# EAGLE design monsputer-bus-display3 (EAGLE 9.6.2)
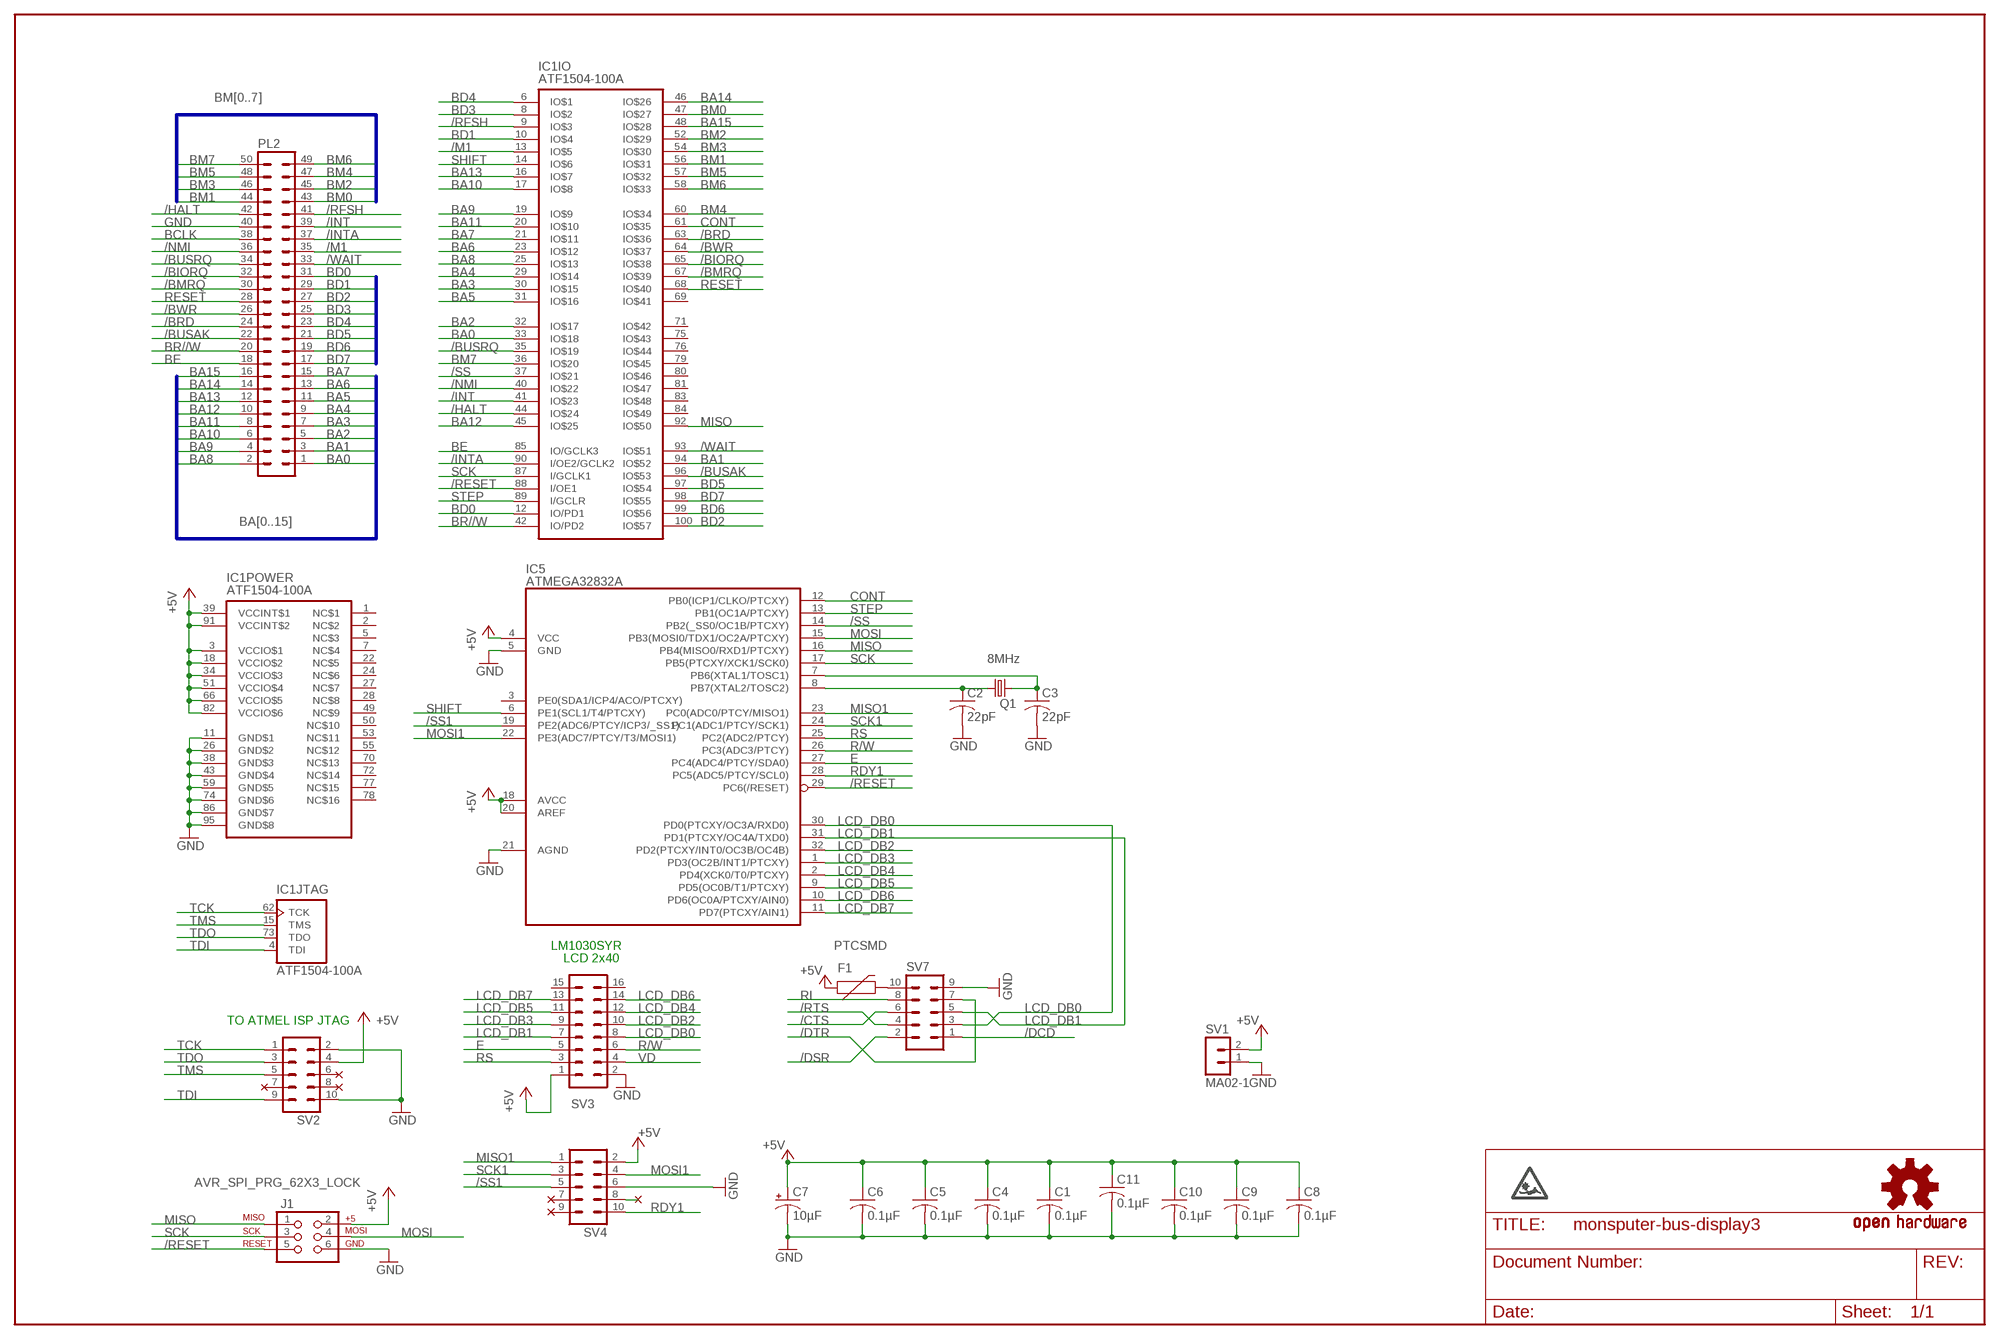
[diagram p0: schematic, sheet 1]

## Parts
C1  0.1µF  C-USC0603  [C0603]
C2  22pF  C-USC0603  [C0603]
C3  22pF  C-USC0603  [C0603]
C4  0.1µF  C-USC0603  [C0603]
C5  0.1µF  C-USC0603  [C0603]
C6  0.1µF  C-USC0603  [C0603]
C7  10µF  CPOL-USCT3528  [CT3528]
C8  0.1µF  C-USC0603  [C0603]
C9  0.1µF  C-USC0603  [C0603]
C10  0.1µF  C-USC0603  [C0603]
C11  0.1µF  C-USC0603  [C0603]
F1  PTCSMD  [PTC-1206]
IC1  ATF1504-100A  [TQFP100]
IC5  ATMEGA32832A  [TQFP32-08]
J1  AVR_SPI_PRG_62X3_LOCK  [2X3_LOCK]
PL2  50H  [50H]
Q1  8MHz  CRYSTALHC49US  [HC49US]
SV1  MA02-1  [MA02-1]
SV2  MA05-2  [MA05-2]
SV3  MA08-2  [MA08-2]
SV4  MA05-2  [MA05-2]
SV7  MA05-2  [MA05-2]
U$1  PHYSNOCT  [PHYSNOCT]
U$2  OSHW-LOGOS  [OSHW-LOGO-S]

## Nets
+5V: C1.1 C4.1 C5.1 C6.1 C7.+ C8.1 C9.1 C10.1 C11.1 F1.1 IC1.3(POWER:VCCIO$1) IC1.18(POWER:VCCIO$2) IC1.34(POWER:VCCIO$3) IC1.39(POWER:VCCINT$1) IC1.51(POWER:VCCIO$4) IC1.66(POWER:VCCIO$5) IC1.82(POWER:VCCIO$6) IC1.91(POWER:VCCINT$2) IC5.4(VCC) IC5.18(AVCC) IC5.20(AREF) J1.2 SV1.2 SV2.4 SV3.1 SV4.2
/BIORQ: IC1.65(IO:IO$38) PL2.32
/BMRQ: IC1.67(IO:IO$39) PL2.30
/BRD: IC1.63(IO:IO$36) PL2.24
/BUSAK: IC1.96(IO:IO$53) PL2.22
/BUSRQ: IC1.35(IO:IO$19) PL2.34
/BWR: IC1.64(IO:IO$37) PL2.26
/CTS: SV7.6
/DCD: SV7.1
/DSR: SV7.2
/DTR: SV7.7
/HALT: IC1.44(IO:IO$24) PL2.42
/INT: IC1.41(IO:IO$23) PL2.39
/INTA: IC1.90(IO:I/OE2/GCLK2) PL2.37
/M1: IC1.13(IO:IO$5) PL2.35
/NMI: IC1.40(IO:IO$22) PL2.36
/RESET: IC1.88(IO:I/OE1) IC5.29(PC6(/RESET)) J1.5
/RFSH: IC1.9(IO:IO$3) PL2.41
/RTS: SV7.4
/SS: IC1.37(IO:IO$21) IC5.14(PB2(_SS0/OC1B/PTCXY))
/SS1: IC5.19(PE2(ADC6/PTCY/ICP3/_SS1)) SV4.5
/WAIT: IC1.93(IO:IO$51) PL2.33
BA0: IC1.33(IO:IO$18) PL2.1
BA1: IC1.94(IO:IO$52) PL2.3
BA2: IC1.32(IO:IO$17) PL2.5
BA3: IC1.30(IO:IO$15) PL2.7
BA4: IC1.29(IO:IO$14) PL2.9
BA5: IC1.31(IO:IO$16) PL2.11
BA6: IC1.23(IO:IO$12) PL2.13
BA7: IC1.21(IO:IO$11) PL2.15
BA8: IC1.25(IO:IO$13) PL2.2
BA9: IC1.19(IO:IO$9) PL2.4
BA10: IC1.17(IO:IO$8) PL2.6
BA11: IC1.20(IO:IO$10) PL2.8
BA12: IC1.45(IO:IO$25) PL2.10
BA13: IC1.16(IO:IO$7) PL2.12
BA14: IC1.46(IO:IO$26) PL2.14
BA15: IC1.48(IO:IO$28) PL2.16
BCLK: PL2.38
BD0: IC1.12(IO:IO/PD1) PL2.31
BD1: IC1.10(IO:IO$4) PL2.29
BD2: IC1.100(IO:IO$57) PL2.27
BD3: IC1.8(IO:IO$2) PL2.25
BD4: IC1.6(IO:IO$1) PL2.23
BD5: IC1.97(IO:IO$54) PL2.21
BD6: IC1.99(IO:IO$56) PL2.19
BD7: IC1.98(IO:IO$55) PL2.17
BE: IC1.85(IO:IO/GCLK3) PL2.18
BM0: IC1.47(IO:IO$27) PL2.43
BM1: IC1.56(IO:IO$31) PL2.44
BM2: IC1.52(IO:IO$29) PL2.45
BM3: IC1.54(IO:IO$30) PL2.46
BM4: IC1.60(IO:IO$34) PL2.47
BM5: IC1.57(IO:IO$32) PL2.48
BM6: IC1.58(IO:IO$33) PL2.49
BM7: IC1.36(IO:IO$20) PL2.50
BR//W: IC1.42(IO:IO/PD2) PL2.20
CONT: IC1.61(IO:IO$35) IC5.12(PB0(ICP1/CLKO/PTCXY))
E: IC5.27(PC4(ADC4/PTCY/SDA0)) SV3.5
GND: C1.2 C2.2 C3.2 C4.2 C5.2 C6.2 C7.- C8.2 C9.2 C10.2 C11.2 IC1.11(POWER:GND$1) IC1.26(POWER:GND$2) IC1.38(POWER:GND$3) IC1.43(POWER:GND$4) IC1.59(POWER:GND$5) IC1.74(POWER:GND$6) IC1.86(POWER:GND$7) IC1.95(POWER:GND$8) IC5.5(GND) IC5.21(AGND) J1.6 PL2.40 SV1.1 SV2.2 SV2.10 SV3.2 SV4.6 SV7.9
LCD_DB0: IC5.30(PD0(PTCXY/OC3A/RXD0)) SV3.8 SV7.3
LCD_DB1: IC5.31(PD1(PTCXY/OC4A/TXD0)) SV3.7 SV7.5
LCD_DB2: IC5.32(PD2(PTCXY/INT0/OC3B/OC4B)) SV3.10
LCD_DB3: IC5.1(PD3(OC2B/INT1/PTCXY)) SV3.9
LCD_DB4: IC5.2(PD4(XCK0/T0/PTCXY)) SV3.12
LCD_DB5: IC5.9(PD5(OC0B/T1/PTCXY)) SV3.11
LCD_DB6: IC5.10(PD6(OC0A/PTCXY/AIN0)) SV3.14
LCD_DB7: IC5.11(PD7(PTCXY/AIN1)) SV3.13
MISO: IC1.92(IO:IO$50) IC5.16(PB4(MISO0/RXD1/PTCXY)) J1.1
MISO1: IC5.23(PC0(ADC0/PTCY/MISO1)) SV4.1
MOSI: IC5.15(PB3(MOSI0/TDX1/OC2A/PTCXY)) J1.4
MOSI1: IC5.22(PE3(ADC7/PTCY/T3/MOSI1)) SV4.4
N$1: F1.2 SV7.10
N$19: SV4.8
N$20: C3.1 IC5.7(PB6(XTAL1/TOSC1)) Q1.2
N$21: C2.1 IC5.8(PB7(XTAL2/TOSC2)) Q1.1
R/W: IC5.26(PC3(ADC3/PTCY)) SV3.6
RDY1: IC5.28(PC5(ADC5/PTCY/SCL0)) SV4.10
RESET: IC1.68(IO:IO$40) PL2.28
RI: SV7.8
RS: IC5.25(PC2(ADC2/PTCY)) SV3.3
SCK: IC1.87(IO:I/GCLK1) IC5.17(PB5(PTCXY/XCK1/SCK0)) J1.3
SCK1: IC5.24(PC1(ADC1/PTCY/SCK1)) SV4.3
SHIFT: IC1.14(IO:IO$6) IC5.6(PE1(SCL1/T4/PTCXY))
STEP: IC1.89(IO:I/GCLR) IC5.13(PB1(OC1A/PTCXY))
TCK: IC1.62(JTAG:TCK) SV2.1
TDI: IC1.4(JTAG:TDI) SV2.9
TDO: IC1.73(JTAG:TDO) SV2.3
TMS: IC1.15(JTAG:TMS) SV2.5
VD: SV3.4
Unconnected: IC1.1(POWER:NC$1) IC1.2(POWER:NC$2) IC1.5(POWER:NC$3) IC1.7(POWER:NC$4) IC1.22(POWER:NC$5) IC1.24(POWER:NC$6) IC1.27(POWER:NC$7) IC1.28(POWER:NC$8) IC1.49(POWER:NC$9) IC1.50(POWER:NC$10) IC1.53(POWER:NC$11) IC1.55(POWER:NC$12) IC1.69(IO:IO$41) IC1.70(POWER:NC$13) IC1.71(IO:IO$42) IC1.72(POWER:NC$14) IC1.75(IO:IO$43) IC1.76(IO:IO$44) IC1.77(POWER:NC$15) IC1.78(POWER:NC$16) IC1.79(IO:IO$45) IC1.80(IO:IO$46) IC1.81(IO:IO$47) IC1.83(IO:IO$48) IC1.84(IO:IO$49) IC5.3(PE0(SDA1/ICP4/ACO/PTCXY)) SV2.6 SV2.7 SV2.8 SV3.15 SV3.16 SV4.7 SV4.9

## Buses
BD[0..7]
BM[0..7]
BA[0..15]

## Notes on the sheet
- LM1030SYR
- LCD 2x40
- TO ATMEL ISP JTAG

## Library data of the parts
C1-C6 C8-C11 = rcl:C-US: CAPACITOR, American symbol
C7 = rcl:CPOL-US: POLARIZED CAPACITOR, American symbol
F1 = SparkFun:PTC: Resettable Fuse PTC
IC1 = newchips:ATF1504-100: Atmel 64-macrocell CPLD
IC5 = newchips2:ATMEGA328: ATmega328PB AVR® Microcontroller with Core Independent Peripherals and PicoPower® Technology
J1 = SparkFun:AVR_SPI_PRG_6: AVR ISP 6 Pin This is the reduced ISP connector for AVR programming. Common on Arduino. This footprint will take up less PCB space and can be used with a 10-pin to 6-pin adapter such as SKU: BOB-08508
PL2 = con-harting-h:50H: CONNECTOR
Q1 = SparkFun:CRYSTAL: Crystals
SV1 = divers:MA02-1: PIN HEADER
SV2 SV4 SV7 = con-lstb:MA05-2: PIN HEADER; OC_FARNELL: unknown; OC_NEWARK: unknown
SV3 = con-lstb:MA08-2: PIN HEADER; OC_FARNELL: unknown; OC_NEWARK: unknown
U$1 = physnoct:PHYSNOCT: Physnoct logo
U$2 = SparkFun:OSHW-LOGO: Open Source Hardware Logo This logo indicates the piece of hardware it is found on incorporates a OSHW license and/or adheres to the definition of open source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

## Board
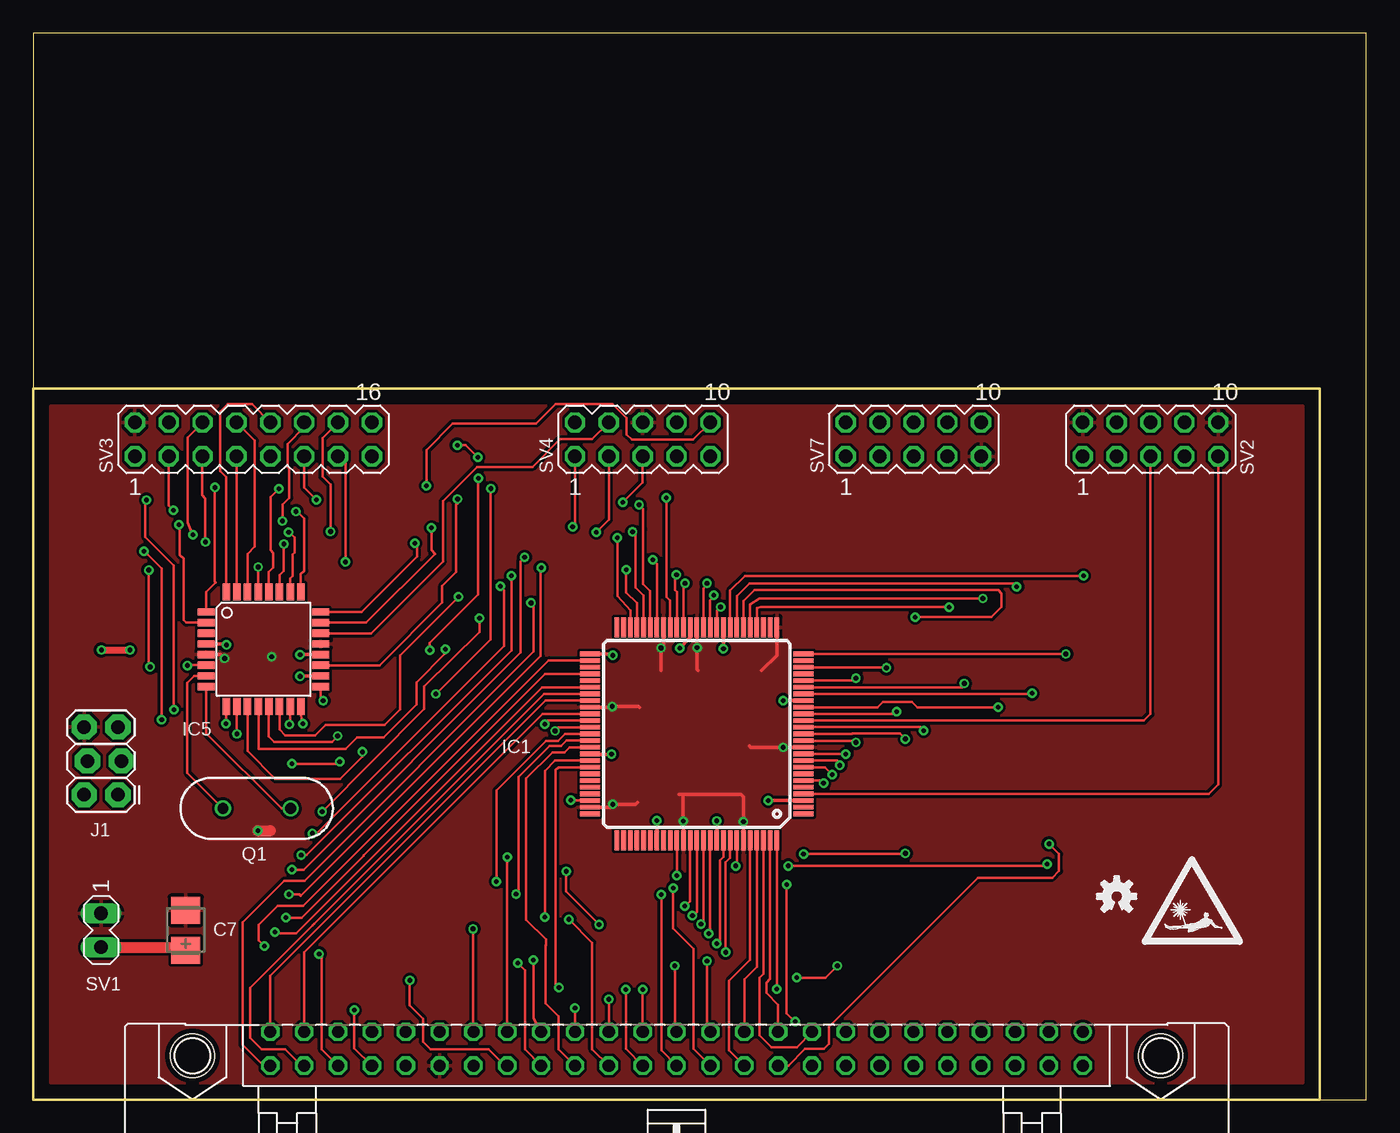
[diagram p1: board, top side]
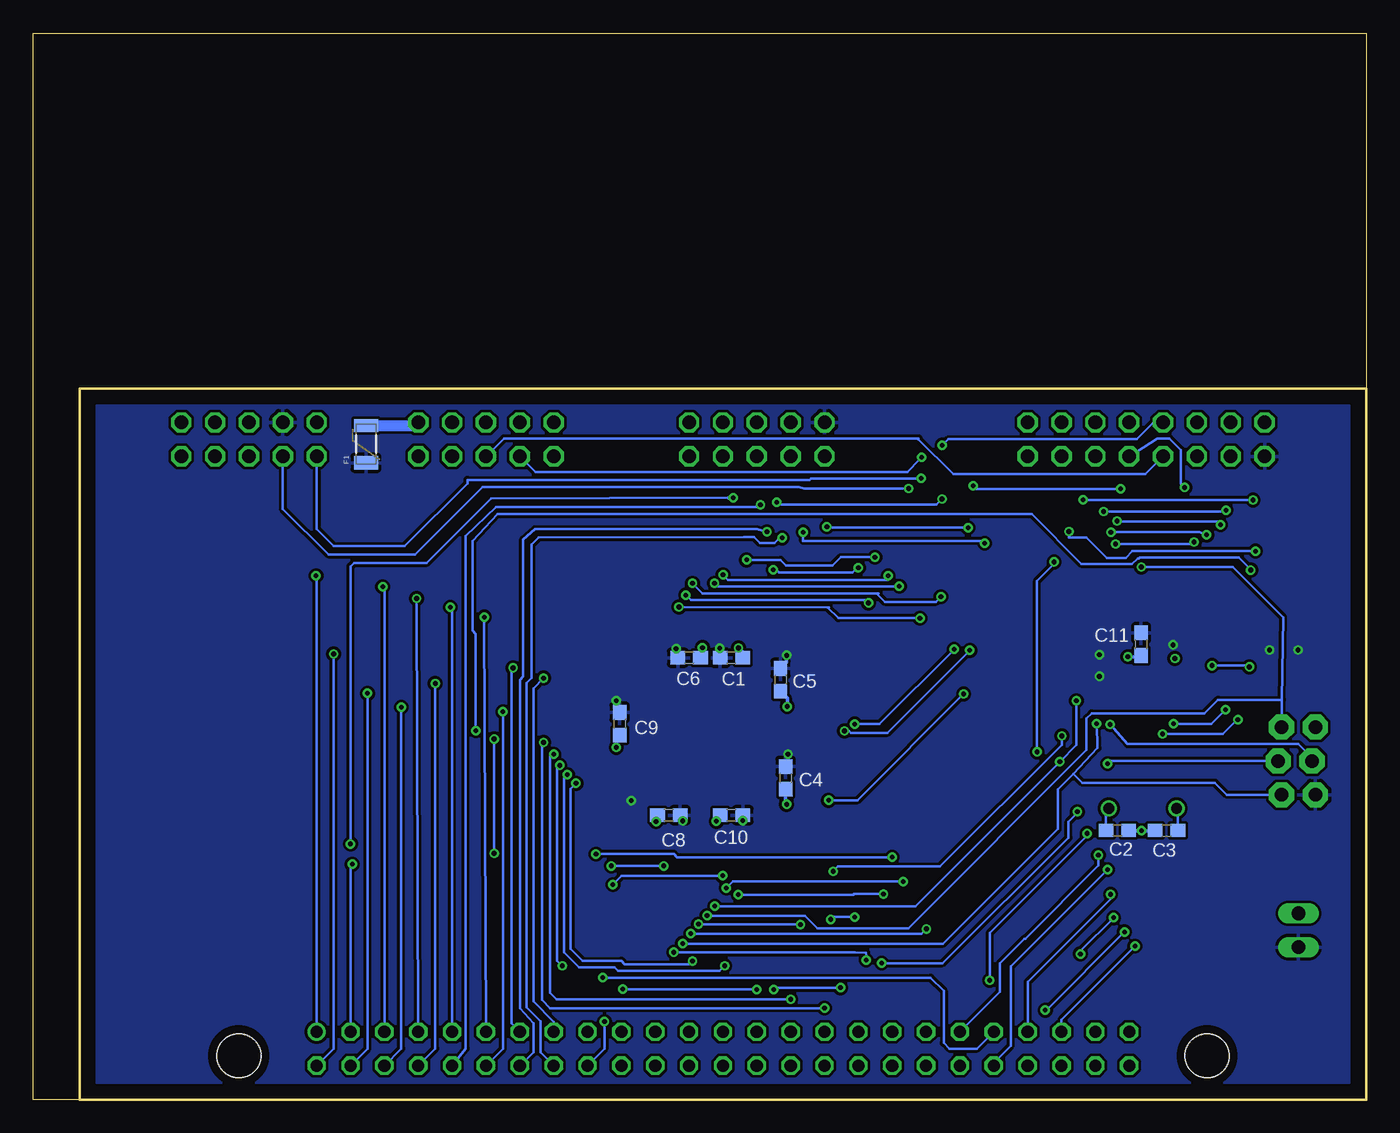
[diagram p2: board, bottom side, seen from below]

Size 100 x 80 mm. Coordinates in mm from the lower left corner, seen from the top.
Outline: 96.52,0 100,0 100,80 0,80 0,53.34
Outline: 0,53.34 0,0 96.52,0
Outline: 0,53.34 96.52,53.34 96.52,0
Copper layers (1*16): Top 0.0356mm / dielectric 1.5011mm / Bottom 0.0356mm
Design rules "OSHPark *": minimum track width 6mil, minimum drill 13mil, track to track 8mil, track to pad 8mil, pad to pad 6mil, via to via 8mil, smd to smd 6mil, copper to edge 15mil, drill to drill 6mil, minimum pad ring 7mil, minimum via ring 7mil, stop-mask expansion 4mil, vias tented up to drill 0mil, thermal gap 10mil

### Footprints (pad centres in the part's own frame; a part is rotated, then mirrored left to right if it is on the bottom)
C0603 = smd 1.1 x 1: 1 -0.85,0; 2 0.85,0
CT3528 = smd 2 x 2.2: + -1.5,0; - 1.5,0
PTC-1206 = smd 1 x 1.8: 1 -1.4,0; 2 1.4,0
TQFP100 = smd 1.5 x 0.35: 1 -8,6; 2 -8,5.5; 3 -8,5; 4 -8,4.5; 5 -8,4; 6 -8,3.5; 7 -8,3; 8 -8,2.5; 9 -8,2; 10 -8,1.5; 11 -8,1; 12 -8,0.5; 13 -8,0; 14 -8,-0.5; 15 -8,-1; 16 -8,-1.5; 17 -8,-2; 18 -8,-2.5; 19 -8,-3; 20 -8,-3.5; 21 -8,-4; 22 -8,-4.5; 23 -8,-5; 24 -8,-5.5; 25 -8,-6; 51 8,-6; 52 8,-5.5; 53 8,-5; 54 8,-4.5; 55 8,-4; 56 8,-3.5; 57 8,-3; 58 8,-2.5; 59 8,-2; 60 8,-1.5; 61 8,-1; 62 8,-0.5; 63 8,0; 64 8,0.5; 65 8,1; 66 8,1.5; 67 8,2; 68 8,2.5; 69 8,3; 70 8,3.5; 71 8,4; 72 8,4.5; 73 8,5; 74 8,5.5; 75 8,6 | smd 0.35 x 1.5: 26 -6,-8; 27 -5.5,-8; 28 -5,-8; 29 -4.5,-8; 30 -4,-8; 31 -3.5,-8; 32 -3,-8; 33 -2.5,-8; 34 -2,-8; 35 -1.5,-8; 36 -1,-8; 37 -0.5,-8; 38 0,-8; 39 0.5,-8; 40 1,-8; 41 1.5,-8; 42 2,-8; 43 2.5,-8; 44 3,-8; 45 3.5,-8; 46 4,-8; 47 4.5,-8; 48 5,-8; 49 5.5,-8; 50 6,-8; 76 6,8; 77 5.5,8; 78 5,8; 79 4.5,8; 80 4,8; 81 3.5,8; 82 3,8; 83 2.5,8; 84 2,8; 85 1.5,8; 86 1,8; 87 0.5,8; 88 0,8; 89 -0.5,8; 90 -1,8; 91 -1.5,8; 92 -2,8; 93 -2.5,8; 94 -3,8; 95 -3.5,8; 96 -4,8; 97 -4.5,8; 98 -5,8; 99 -5.5,8; 100 -6,8
TQFP32-08 = smd 1.27 x 0.559: 1 -4.293,2.8; 2 -4.293,2; 3 -4.293,1.2; 4 -4.293,0.4; 5 -4.293,-0.4; 6 -4.293,-1.2; 7 -4.293,-2; 8 -4.293,-2.8; 17 4.293,-2.8; 18 4.293,-2; 19 4.293,-1.2; 20 4.293,-0.4; 21 4.293,0.4; 22 4.293,1.2; 23 4.293,2; 24 4.293,2.8 | smd 0.559 x 1.27: 9 -2.8,-4.293; 10 -2,-4.293; 11 -1.2,-4.293; 12 -0.4,-4.293; 13 0.4,-4.293; 14 1.2,-4.293; 15 2,-4.293; 16 2.8,-4.293; 25 2.8,4.293; 26 2,4.293; 27 1.2,4.293; 28 0.4,4.293; 29 -0.4,4.293; 30 -1.2,4.293; 31 -2,4.293; 32 -2.8,4.293
2X3_LOCK = drill 1.016 pad 1.88 octagon: 1 0,0; 2 0,2.54; 3 2.54,-0.254; 4 2.54,2.286; 5 5.08,0; 6 5.08,2.54
50H = drill 0.914: 1 -30.48,-1.27 | drill 0.914 octagon: 2 -30.48,1.27; 3 -27.94,-1.27; 4 -27.94,1.27; 5 -25.4,-1.27; 6 -25.4,1.27; 7 -22.86,-1.27; 8 -22.86,1.27; 9 -20.32,-1.27; 10 -20.32,1.27; 11 -17.78,-1.27; 12 -17.78,1.27; 13 -15.24,-1.27; 14 -15.24,1.27; 15 -12.7,-1.27; 16 -12.7,1.27; 17 -10.16,-1.27; 18 -10.16,1.27; 19 -7.62,-1.27; 20 -7.62,1.27; 21 -5.08,-1.27; 22 -5.08,1.27; 23 -2.54,-1.27; 24 -2.54,1.27; 25 0,-1.27; 26 0,1.27; 27 2.54,-1.27; 28 2.54,1.27; 29 5.08,-1.27; 30 5.08,1.27; 31 7.62,-1.27; 32 7.62,1.27; 33 10.16,-1.27; 34 10.16,1.27; 35 12.7,-1.27; 36 12.7,1.27; 37 15.24,-1.27; 38 15.24,1.27; 39 17.78,-1.27; 40 17.78,1.27; 41 20.32,-1.27; 42 20.32,1.27; 43 22.86,-1.27; 44 22.86,1.27; 45 25.4,-1.27; 46 25.4,1.27; 47 27.94,-1.27; 48 27.94,1.27; 49 30.48,-1.27; 50 30.48,1.27 | hole 3.302: -36.322,0.533; 36.322,0.533
HC49US = drill 0.813: 1 -2.54,0; 2 2.54,0
MA02-1 = drill 1.016 long: 1 -2.54,0; 2 0,0
MA05-2 = drill 1.016 octagon: 1 -5.08,-1.27; 2 -5.08,1.27; 3 -2.54,-1.27; 4 -2.54,1.27; 5 0,-1.27; 6 0,1.27; 7 2.54,-1.27; 8 2.54,1.27; 9 5.08,-1.27; 10 5.08,1.27
MA08-2 = drill 1.016 octagon: 1 -8.89,-1.27; 2 -8.89,1.27; 3 -6.35,-1.27; 4 -6.35,1.27; 5 -3.81,-1.27; 6 -3.81,1.27; 7 -1.27,-1.27; 8 -1.27,1.27; 9 1.27,-1.27; 10 1.27,1.27; 11 3.81,-1.27; 12 3.81,1.27; 13 6.35,-1.27; 14 6.35,1.27; 15 8.89,-1.27; 16 8.89,1.27

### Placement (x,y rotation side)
C1  47.62,33.15 0 bottom
C2  18.67,20.19 0 bottom
C3  14.99,20.19 180 bottom
C4  43.56,24.13 270 bottom
C5  43.94,31.5 270 bottom
C6  50.8,33.15 0 bottom
C7  11.43,12.7 90 top
C8  52.32,21.34 180 bottom
C9  56.01,28.19 270 bottom
C10  47.62,21.34 180 bottom
C11  16.89,34.16 270 bottom
F1  75.03,49.17 90 bottom
IC1  49.78,27.43 180 top
IC5  17.27,33.78 0 top
J1  6.35,22.86 90 top
PL2  48.26,3.81 180 top
Q1  16.76,21.84 180 top
SV1  5.08,11.43 270 top
SV2  83.82,49.53 0 top
SV3  16.51,49.53 0 top
SV4  45.72,49.53 0 top
SV7  66.04,49.53 0 top
U$1  83.11,11.53 0 top
U$2  81.28,15.24 0 top

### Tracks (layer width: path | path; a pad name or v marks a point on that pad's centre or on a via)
+5V  (via drill 0.35)
  Top 0.254: IC1.3 v55.15,22.43 v55.14,22.43 | IC1.39 49.28,34.65 v48.49,33.86 | IC1.34 v51.78,33.84 v51.78,33.83 | IC1.18 v56.26,29.93 | IC1.91 51.28,20.89 v51.27,20.9 | IC1.82 46.78,20.92 v46.77,20.93 | IC1.66 41.81,25.91 v43.38,25.91 | IC1.51 43.38,33.43 v43.48,33.33 | IC5.20 v20.02,33.38 | IC5.18 20.05,31.78 v20.02,31.75 | IC5.4 14.41,34.18 v14.48,34.11
  Top 0.508: v5.11,33.73 v7.24,33.73
  Top 0.813: SV1.2 11.2,11.43 C7.+
  Bottom 0.254: v48.49,33.86 48.49,33.16 C1.1 | C6.1 51.78,33.27 v51.78,33.83 | C9.1 56.26,29.3 v56.26,29.93 | C8.1 51.47,21.11 v51.27,20.9 | C10.1 v46.77,20.93 | C4.1 43.38,25.16 v43.38,25.91 | C5.1 43.48,32.8 v43.48,33.33
  pour Bottom: 44.2,33.15 55.63,33.15 55.63,21.46 44.2,21.59
  pour Bottom: 1.27,1.27 1.27,52.07 95.25,52.07 95.25,1.27
/BIORQ
  Top 0.203: PL2.32 39.4,3.79 39.4,6.25 38.43,7.21 38.43,11.56 38.46,11.58 38.46,12.01 36.98,13.49 36.98,24.08 38.96,26.06 39.85,26.06 40.22,26.43 IC1.65
/BMRQ  (via drill 0.35)
  Top 0.203: IC1.67 39.15,25.43 38.38,24.66 v38.38,13.69 | PL2.30 41.94,3.79 41.94,11.76 v40.18,13.51
  Bottom 0.203: v40.18,13.51 40.01,13.69 v38.38,13.69
/BRD  (via drill 0.35)
  Top 0.203: IC1.63 39.88,27.43 39.37,26.92 38.48,26.92 34.75,23.19 v34.75,16.36 | PL2.24 49.53,3.81 49.53,11.3 48.01,12.83 v48.01,15.88
  Bottom 0.203: v48.01,15.88 47.5,16.38 34.77,16.38 v34.75,16.36
/BUSAK
  Top 0.203: IC1.96 53.78,10.48 52.2,8.89 52.2,3.68 PL2.22
/BUSRQ  (via drill 0.35)
  Top 0.203: IC1.35 51.28,36.68 v51.56,36.96 | PL2.34 36.88,3.76 36.88,9.7 v36.35,10.24 | v21.67,21.59 29.34,29.31 29.34,30.99 33.48,35.08 v33.48,36.12
  Bottom 0.203: v51.56,36.96 40.41,36.93 | 40.41,36.93 40.31,36.93 | v36.35,10.24 31.8,10.24 22.33,19.63 22.33,20.83 21.67,21.49 v21.67,21.59 | v33.48,36.12 39.6,36.12 40.41,36.93
/BWR  (via drill 0.35)
  Top 0.203: PL2.26 47.12,3.68 v47.12,15.37 | IC1.64 40.01,26.93 39.6,26.52 38.73,26.52 36.42,24.21 36.42,15.62 v36.22,15.42
  Bottom 0.203: v47.12,15.37 38.48,15.37 38.43,15.42 v36.22,15.42
/HALT  (via drill 0.35)
  Top 0.203: v46.48,40.49 46.78,40.19 IC1.44 | v19.41,17.25 20.27,17.25 36.55,33.53 36.55,40.39 v36.85,40.69
  Bottom 0.203: v46.48,40.49 43.94,40.49 43.54,40.08 40.03,40.08 39.42,40.69 v36.85,40.69 | PL2.42 27.94,2.77 26.67,4.04 26.67,9.98 v19.41,17.25
/INT  (via drill 0.35)  (1 unrouted)
  Top 0.203: IC1.41 48.28,38.08 48.13,38.23 48.13,39.24 v48.26,39.37 v48.25,39.38 | v20.09,18.34 20.52,18.34 35.87,33.68 v35.87,39.29
  Bottom 0.203: v48.25,39.38 47.86,38.99 35.89,38.99 v35.87,39.29 | PL2.39 27.48,8.08 27.48,10.21 25.63,12.06 25.58,12.06 20.09,17.55 v20.09,18.34
/INTA  (via drill 0.35)
  Top 0.203: IC1.90 50.78,12.56 v50.67,12.45 | v32.99,12.8 32.99,5.11 PL2.37
  Bottom 0.203: v32.99,12.8 33.35,12.45 v50.67,12.45
/M1  (via drill 0.35)
  Top 0.203: IC1.13 61.43,27.43 61.45,27.45 65,27.45 65.41,27.05 v65.43,27.05 | PL2.35 v35.56,18.19 | v57.78,18.41 65.35,18.41 65.41,18.47 v65.43,18.47
  Bottom 0.203: v35.56,18.19 51.69,18.19 51.94,18.44 57.63,18.44 57.68,18.39 57.76,18.39 v57.78,18.41 | v65.43,18.47 v65.43,27.05
/NMI  (via drill 0.35)
  Top 0.203: IC1.40 48.78,38.62 v48.9,38.73 | PL2.36 35.41,2.54 34.16,3.79 29.79,3.79 29.23,4.34 29.23,6.07 28.25,7.06 v28.25,8.94 | v20.93,19.96 21.26,19.96 35.33,34.04 35.33,38.18 35.03,38.48 v35.03,38.51
  Bottom 0.203: v48.9,38.73 48.77,38.61 48.77,38.48 36.64,38.48 36.62,38.51 v35.03,38.51 | v28.25,8.94 28.25,12.5 20.93,19.81 v20.93,19.96
/RESET  (via drill 0.35)
  Top 0.203: IC1.88 49.78,14.1 49.53,13.84 v49.45,13.79 | v16.87,39.95 16.87,40.06 IC5.29
  Bottom 0.203: v49.45,13.79 42.12,13.79 41.18,12.86 34.34,12.86 20.98,26.21 20.98,28.6 20.6,28.98 12.14,28.98 11.12,30 6.32,30 | J1.5 6.32,30 | 6.32,30 6.22,36.17 10.01,39.95 v16.87,39.95 16.79,39.98
/RFSH  (via drill 0.35)
  Top 0.203: 57.8,25.41 IC1.9 60.29,25.43 60.58,25.15 v60.51,25.07 | v60.33,10.03 59.44,9.14 v57.28,9.14
  Bottom 0.203: v60.51,25.07 60.71,24.88 60.71,10.41 v60.33,10.03 | v57.28,9.14 32.69,9.14 31.7,8.15 31.7,4.24 31.27,3.81 29.21,3.81 PL2.41
/SS  (via drill 0.35)
  Top 0.203: IC1.37 50.28,38.35 50.55,38.61 v50.55,38.73 | IC5.14 18.47,27.76 18.9,27.33 21.16,27.33 21.92,28.09 26.34,28.09 27.51,29.26 27.51,33.33 v31.9,37.72
  Bottom 0.203: v50.55,38.73 49.78,37.97 36.75,37.97 | 36.75,37.97 36.58,37.97 | 36.75,37.97 36.12,37.34 32.28,37.34 v31.9,37.72
/SS1  (via drill 0.35)
  Top 0.203: IC5.19 25.98,32.58 30.68,37.29 30.68,38.53 31.73,39.57 31.73,44.63 31.83,44.73 v31.83,45.06 | v44.22,44.81 45.72,46.3 SV4.5
  Bottom 0.203: v31.83,45.06 32.23,44.65 44.07,44.65 v44.22,44.81
/WAIT  (via drill 0.35)
  Top 0.203: IC1.93 52.28,18.12 51.94,17.78 v51.94,11.05 | v37.52,10.46 37.54,6.1 PL2.33
  Bottom 0.203: v51.94,11.05 38.51,11.05 | 38.51,11.05 38.35,11.05 | 38.51,11.05 37.52,11.02 37.47,10.54 v37.52,10.46
BA0  (via drill 0.35)
  Top 0.203: IC1.33 52.28,38.19 53.39,39.29 v78.79,39.29
  Bottom 0.203: PL2.1 78.74,39.24 v78.79,39.29
BA1  (via drill 0.35)
  Top 0.203: IC1.94 52.78,17.61 v52.7,17.53 | v56.64,17.53 75.95,17.53 v76.07,17.65
  Bottom 0.203: v52.7,17.53 v56.64,17.53 | PL2.3 76.2,17.53 v76.07,17.65
BA2  (via drill 0.35)
  Top 0.203: IC1.32 52.78,37.8 53.72,38.73 73.53,38.73 v73.79,38.48
  Bottom 0.203: PL2.5 73.66,38.35 v73.79,38.48
BA3  (via drill 0.35)
  Top 0.203: IC1.30 53.78,37.15 54.48,37.59 v71.25,37.59
  Bottom 0.203: PL2.7 v71.25,37.59
BA4  (via drill 0.35)
  Top 0.203: IC1.29 54.28,36.88 54.61,36.96 68.71,36.96 v68.71,36.93
  Bottom 0.203: PL2.9 68.58,37.08 68.71,37.21 v68.71,36.93
BA5  (via drill 0.35)
  Top 0.203: IC1.31 53.28,37.41 54.1,38.23 70.95,38.23 70.97,38.25 71.52,38.25 71.54,38.23 72.39,38.23 72.64,37.97 72.64,36.96 71.88,36.2 v66.17,36.2
  Bottom 0.203: PL2.11 v66.17,36.2
BA6  (via drill 0.35)
  Top 0.203: IC1.23 63.58,32.43 v64.01,32.38
  Bottom 0.203: PL2.13 64.14,5.71 64.14,28.8 64.11,28.82 64.11,32.15 64.01,32.26 v64.01,32.38
BA7  (via drill 0.35)
  Top 0.203: IC1.21 61.53,31.43 v61.72,31.62
  Bottom 0.203: PL2.15 60.96,5.84 62.48,7.37 62.48,30.86 v61.72,31.62
BA8  (via drill 0.35)
  Top 0.203: IC1.25 v77.47,33.43
  Bottom 0.203: PL2.2 77.47,3.81 v77.47,33.43
BA9  (via drill 0.35)
  Top 0.203: v74.93,30.48 74.88,30.43 IC1.19
  Bottom 0.203: PL2.4 74.93,3.81 v74.93,30.48
BA10  (via drill 0.35)
  Top 0.203: IC1.17 63.34,29.43 63.75,29.84 65.91,29.84 66.33,29.43 v72.39,29.43
  Bottom 0.203: PL2.6 72.39,3.81 v72.39,29.43 72.39,29.46
BA11  (via drill 0.35)
  Top 0.203: IC1.20 69.72,30.93 69.85,31.06 v69.85,31.22
  Bottom 0.203: PL2.8 69.85,3.81 v69.85,31.22 69.85,31.37
BA12  (via drill 0.35)
  Top 0.203: IC1.45 46.28,38.15 45.74,38.68 45.74,42.8 45.74,44.32 v45.44,44.63
  Bottom 0.203: PL2.10 67.56,3.81 67.56,42.29 65.28,44.45 45.67,44.45 45.49,44.63 v45.44,44.63
BA13  (via drill 0.35)
  Top 0.203: v64.77,29.09 64.61,28.93 IC1.16
  Bottom 0.203: PL2.12 64.77,3.81 v64.77,29.09
BA14  (via drill 0.35)
  Top 0.203: IC1.46 45.78,37.83 45.19,38.43 45.19,42.37 v44.96,42.6
  Bottom 0.203: PL2.14 62.48,3.56 62.48,5.71 63.5,6.86 63.5,31.5 63.25,31.75 63.25,42.04 62.36,42.8 45.72,42.8 v44.96,42.6
BA15  (via drill 0.35)
  Top 0.203: IC1.48 44.8,35.45 44.8,36.31 44.81,36.31 44.81,36.7 43.81,37.8 v43.81,42.14
  Bottom 0.203: PL2.16 61.95,3.53 61.95,5.88 62.99,6.92 62.99,31.24 62.61,31.62 62.61,41.66 62.1,42.16 46.69,42.19 45.92,42.19 45.49,41.76 44.4,41.76 44.07,42.09 v43.81,42.14
BD0  (via drill 0.35)
  Top 0.203: IC1.12 57.79,26.92 61.59,26.92 v61.72,26.8 | PL2.31 v40.64,6.86
  Bottom 0.203: v61.72,26.8 61.85,26.67 61.85,7.49 61.21,6.86 v40.64,6.86
BD1  (via drill 0.35)
  Top 0.203: IC1.10 60.94,25.93 v60.96,25.91 | PL2.29 v43.18,7.52
  Bottom 0.203: v60.96,25.91 61.21,25.91 61.21,8 60.73,7.52 v43.18,7.52
BD2  (via drill 0.35)
  Top 0.203: PL2.27 v45.72,8.26 | IC1.100 v55.78,8.29 55.75,8.26
  Bottom 0.203: v45.72,8.26 55.75,8.26 v55.78,8.29
BD3  (via drill 0.35)
  Top 0.203: IC1.8 59.4,24.93 59.94,24.38 v59.93,24.37 | v48.13,10.03 48.13,5.21 PL2.25
  Bottom 0.203: v59.93,24.37 60.2,24.1 60.2,11.05 59.05,9.91 56.39,9.91 56.13,9.65 48.51,9.65 v48.13,10.03
BD4  (via drill 0.35)
  Top 0.203: IC1.6 59.13,23.93 59.31,23.75 v59.29,23.73 | v50.55,10.39 50.55,5.33 PL2.23
  Bottom 0.203: v59.29,23.73 59.69,23.32 59.69,11.3 58.8,10.41 55.88,10.41 55.63,10.16 50.8,10.16 50.55,10.41 v50.55,10.39
BD5
  Top 0.203: IC1.97 54.28,9.96 53.34,9.02 PL2.21
BD6
  Top 0.203: IC1.99 55.28,9.06 54.99,8.76 54.99,8 55.88,7.11 PL2.19
BD7
  Top 0.203: IC1.98 54.78,9.45 54.48,9.14 54.48,4.83 55.37,3.94 57.28,3.94 PL2.17
BE  (via drill 0.35)
  Top 0.203: IC1.85 v48.28,16.79 48.26,16.76 | v56.52,16.13 56.52,6.48 v57.15,5.84
  Bottom 0.203: v48.28,16.79 55.86,16.79 v56.52,16.13 | v57.15,5.84 57.15,3.81 PL2.18
BM0  (via drill 0.35)
  Top 0.203: IC1.47 45.28,37.24 44.48,38.05 v44.48,39.75 | v19.18,15.39 19.96,15.39 20.07,15.29 38.05,33.27 38.08,33.27 38.08,39.65 38.2,39.78 38.1,39.88 v38.1,39.9
  Bottom 0.203: v44.48,39.75 44.25,39.75 44.04,39.55 38.53,39.55 38.18,39.9 v38.1,39.9 | PL2.43 25.4,8.81 19.07,15.14 19.18,15.24 v19.18,15.39
BM1  (via drill 0.35)
  Top 0.203: IC1.56 38.17,30.93 19.71,12.47 18.11,12.47 18.11,12.55 v18.14,12.57 | v24.08,6.71 24.08,3.86 PL2.44
  Bottom 0.203: v18.14,12.57 24,6.71 v24.08,6.71
BM2  (via drill 0.35)
  Top 0.203: IC1.52 38.65,32.93 20.24,14.53 18.34,14.53 16.92,13.11 16.92,11.94 v17.35,11.51
  Bottom 0.203: v17.35,11.51 22.86,5.99 PL2.45
BM3  (via drill 0.35)
  Top 0.203: IC1.54 38.41,31.93 24.79,18.31 24.77,18.29 20.12,13.64 v18.95,13.64 | PL2.46 21.64,3.76 21.64,10.72 v21.44,10.92
  Bottom 0.203: v21.44,10.92 21.44,11.15 v18.95,13.64
BM4
  Top 0.203: IC1.60 38.2,28.93 20.32,11.05 PL2.47
BM5
  Top 0.203: IC1.57 38.31,30.43 21.06,13.18 20.95,13.08 16.26,8.38 16.26,4.65 17.12,3.79 18.9,3.79 20.14,2.54 PL2.48
BM6
  Top 0.203: IC1.58 38.44,29.93 17.78,9.27 PL2.49
BM7  (via drill 0.35)
  Top 0.203: IC1.36 50.78,37.45 50.93,37.59 v51.05,37.85 | PL2.50 17.7,2.62 17.2,2.62 15.7,4.12 15.7,13.28 18.82,16.41 20.34,16.41 37.54,33.6 37.54,35.64 | 37.54,35.64 37.52,35.66 | v37.34,37.26 37.34,37.24 37.54,36.96 37.54,35.64
  Bottom 0.203: v51.05,37.85 50.67,37.47 37.62,37.49 37.39,37.29 v37.34,37.26
BR//W  (via drill 0.35)
  Top 0.203: IC1.42 47.78,37.43 47.5,37.72 v47.5,45.16 | PL2.20 56.64,2.54 57.91,3.81 59.31,3.81 59.69,4.19 59.69,5.46 70.87,16.64 76.45,16.64 76.96,17.14 76.96,18.41 v76.2,19.18
  Bottom 0.203: v76.2,19.18 76.2,40.01 75.95,40.26 70.48,40.26 65.66,45.09 47.88,45.19 47.86,45.11 v47.5,45.16
CONT  (via drill 0.35)
  Top 0.203: IC1.61 38.59,28.43 38.35,28.19 v38.37,28.17 | IC5.12 16.89,29.47 16.89,26.29 23.42,26.29 24.28,27.15 26.26,27.15 28.75,29.64 28.75,31.29 30.91,33.45 v30.91,33.78
  Bottom 0.203: v30.91,33.78 36.52,28.17 v38.37,28.17
E  (via drill 0.35)
  Top 0.203: IC5.27 18.47,39.35 18.8,39.67 v18.8,41.68 | v12.9,41.83 12.9,45.11 12.68,45.34 12.68,48.23 SV3.5
  Bottom 0.203: v18.8,41.68 13.13,41.68 12.85,41.96 v12.9,41.83
GND  (via drill 0.35)
  Top 0.254: 48.82,22.91 53.09,22.91 53.28,22.72 v53.28,20.85 v53.28,20.84 IC1.95 | 48.82,22.91 48.44,22.91 | IC1.26 55.78,33.33 54.63,32.18 | IC1.38 49.78,33.92 v49.8,33.91 49.8,32.27 49.86,32.21 | IC1.43 47.28,34.08 v47.09,33.88 47.09,32.18 | IC1.11 56.28,26.43 v56.26,26.42 53.82,26.42 53.72,26.52 | IC1.86 48.78,20.85 v48.75,20.88 48.75,22.85 48.82,22.91 | IC1.74 43.27,21.93 v43.48,22.15 45.19,22.15 45.31,22.28 | IC1.59 43.38,29.43 v43.43,29.49 45.41,29.49 45.49,29.41 | IC5.5 14.06,33.38 v14.35,33.1
  Top 0.813: v16.84,20.17 17.75,20.17 17.78,20.19
  Bottom 0.254: 56.06,27.29 C9.2 56.26,27.09 v56.26,26.42 | v49.8,33.91 49.8,33.3 C6.2 | C1.2 46.77,33.57 v47.09,33.88 | C8.2 53.17,20.95 v53.28,20.85 | C10.2 48.48,21.16 v48.75,20.88 | C4.2 43.56,22.23 v43.48,22.15 | C5.2 43.43,30.14 v43.43,29.49 | v17.88,33.22 16.98,33.22 C11.2 | C2.2 17.79,20.17 v16.84,20.17 15.86,20.17 C3.2
  pour Top: 44.2,33.15 55.63,33.15 55.63,21.46 44.2,21.46
  pour Top: 1.32,1.27 1.32,52.04 95.25,52.04 95.25,1.27 92.99,1.27 92.96,1.3 92.94,1.27
LCD_DB0  (via drill 0.35)
  Top 0.203: IC5.30 16.07,40.94 16.61,41.48 16.61,49.43 SV3.8 | v33.35,48.18 32.44,49.1 v31.8,49.1
  Bottom 0.203: SV7.3 62.33,47.09 34.42,47.09 33.5,48.01 33.5,48.03 v33.35,48.18 | v31.8,49.1 31.34,49.55 17.22,49.55 15.98,50.8 SV3.8
LCD_DB1
  Top 0.203: SV3.7 15.24,38.11 IC5.31
  Bottom 0.203: SV3.7 16.59,46.91 30.96,46.91 33.58,49.53 33.58,49.61 64.69,49.61 SV7.5
LCD_DB2
  Top 0.203: IC5.32 14.47,46.69 14.02,47.14 14.02,51.61 14.58,52.17 16.41,52.17 SV3.10
LCD_DB3  (via drill 0.35)
  Top 0.203: v13.61,45.92 13.61,38.86 13.69,38.79 12.98,38.08 IC5.1
  Bottom 0.203: 17.78,48.16 SV3.9 15.67,49.61 14.76,49.61 13.89,48.74 13.89,46.2 v13.61,45.92
LCD_DB4  (via drill 0.35)
  Top 0.203: SV3.12 20.32,50.44 19.07,49.2 19.07,47.47 19.2,47.35 19.2,45.14 18.7,44.63 v18.7,43.4 | IC5.2 11.49,35.78 11.28,35.99 11.28,40.59 11,40.87 11,43.13 v10.93,43.13
  Bottom 0.203: v10.93,43.13 11.18,43.38 18.69,43.38 18.7,43.38 | 18.72,43.36 18.7,43.38 | 18.7,43.38 v18.7,43.4
LCD_DB5  (via drill 0.35)
  Top 0.203: IC5.9 14.47,28.21 v14.45,28.19 | v10.54,29.26 10.54,40.06 8.41,42.19 8.41,44.91 v8.48,44.98 | v21.23,45.01 20.32,45.92 SV3.11
  Bottom 0.203: v14.45,28.19 11.61,28.19 v10.54,29.26 | v21.23,45.01 21.21,44.98 v8.48,44.98
LCD_DB6  (via drill 0.35)
  Top 0.203: IC5.10 v15.27,27.44 v15.27,27.43 | v9.63,28.5 9.63,39.83 v8.31,41.15 | v22.3,42.62 22.3,46.13 21.69,46.74 21.69,49.63 SV3.14
  Bottom 0.203: v15.27,27.43 10.77,27.43 9.68,28.52 9.65,28.5 v9.63,28.5 | v8.31,41.15 17.53,41.15 18.03,40.64 19.46,40.64 20.98,42.16 22.3,42.16 v22.3,42.62
LCD_DB7  (via drill 0.35)
  Top 0.203: IC5.11 16.07,26.14 18.16,24.05 23.01,24.05 24.69,25.73 v24.69,26.09 | v23.42,40.34 23.42,47.7 SV3.13
  Bottom 0.203: v24.69,26.09 24.69,38.91 23.42,40.18 v23.42,40.34
MISO  (via drill 0.35)
  Top 0.203: IC1.92 51.78,18.2 51.54,17.95 51.54,11.91 51.31,11.68 v51.28,11.71 | v20.22,28.19 20.12,28.44 IC5.16
  Bottom 0.203: v51.28,11.71 51.26,11.68 31.75,11.68 23.14,20.3 23.14,23.27 21.96,24.45 | 21.96,24.45 20.17,26.36 v20.22,28.19 | J1.1 10.44,22.86 11.35,23.77 21.29,23.77 21.96,24.45
MISO1  (via drill 0.35)
  Top 0.203: IC5.23 24.99,35.78 30.15,40.95 29.87,41.22 v29.87,42.9 | v40.46,42.98 40.64,43.16 SV4.1
  Bottom 0.203: v29.87,42.9 40.39,42.9 v40.46,42.98
MOSI  (via drill 0.35)
  Top 0.203: IC5.15 19.27,28.04 v19.2,28.14
  Bottom 0.203: v19.2,28.14 17.91,26.67 5.08,26.67 4.06,25.65 J1.4
MOSI1
  Top 0.203: IC5.22 25.33,34.98 30.73,40.39 30.73,44.9 33.31,47.47 37.44,47.47 39.5,49.53 39.5,49.55 41.94,49.55 SV4.4
N$1
  Bottom 0.813: F1.2 71.35,50.57 SV7.10
N$20
  Top 0.203: IC5.7 12.07,31.78 11.56,31.27 11.56,24.51 Q1.2
  Bottom 0.203: C3.1 14.14,21.76 Q1.2
N$21
  Top 0.203: IC5.8 12.98,27.48 18.62,21.84 Q1.1
  Bottom 0.203: C2.1 19.52,21.63 Q1.1
R/W  (via drill 0.35)
  Top 0.203: IC5.26 19.27,39.11 19.46,39.29 19.46,40.89 19.61,41.05 19.61,42.16 19.2,42.57 19.15,42.55 19.18,42.57 v19.15,42.57 | v11.96,42.37 11.58,43.31 11.58,49.68 SV3.6
  Bottom 0.203: v19.15,42.57 12.52,42.6 v11.96,42.37
RDY1  (via drill 0.35)
  Top 0.203: IC5.28 17.67,39.57 18.01,39.9 18.01,41.02 17.8,41.22 17.8,45.21 v18.41,45.82 | SV4.10 49.51,49.51 44.91,49.51 44.5,49.91 44.5,51.13 43.46,52.17 39.17,52.17 37.72,50.72 31.47,50.72 29.49,48.74 v29.49,46.05
  Bottom 0.203: v29.49,46.05 29.26,45.82 v18.41,45.82
RESET  (via drill 0.35)
  Top 0.203: PL2.28 44.45,3.81 v44.45,8.26 | IC1.68 39.41,24.93 39.19,24.71 39.19,8.56 39.27,8.56 v39.44,8.39
  Bottom 0.203: v44.45,8.26 44.31,8.39 v39.44,8.39
RS  (via drill 0.35)
  Top 0.203: IC5.25 20.07,39.43 20.32,39.67 20.32,43.61 19.71,44.22 v19.71,44.12 | v10.52,44.22 10.16,44.58 SV3.3
  Bottom 0.203: v19.71,44.12 10.62,44.12 v10.52,44.22
SCK  (via drill 0.35)
  Top 0.203: IC1.87 49.28,14.87 49.02,14.61 v48.87,14.5 | v19.41,25.2 22.84,25.2 v22.99,25.35 | v21.74,29.92 21.57,30.1 IC5.17
  Bottom 0.203: J1.3 19.2,25.4 v19.41,25.2 | v21.74,29.92 21.74,26.59 v22.99,25.35 33.84,14.5 v48.87,14.5
SCK1  (via drill 0.35)
  Top 0.203: IC5.24 24.62,36.58 28.78,40.74 28.78,41.58 v28.63,41.73 | v42.24,42.57 43.18,43.51 SV4.3
  Bottom 0.203: v28.63,41.73 28.8,41.91 42.24,41.91 v42.24,42.57
SHIFT  (via drill 0.35)
  Top 0.203: IC1.14 57.79,27.94 66.55,27.94 v66.8,27.69 | IC5.6 11.56,32.59 v11.56,32.56 | v8.66,39.73 8.66,32.56 v8.76,32.46
  Bottom 0.203: v66.8,27.69 66.8,34.92 67.06,35.18 67.06,41.91 65.18,43.92 25.09,43.92 21.36,40.18 17.57,40.18 17.14,40.61 17.05,40.61 16.99,40.66 9.55,40.66 8.61,39.73 v8.66,39.73 | v11.56,32.56 8.87,32.56 v8.76,32.46
STEP  (via drill 0.35)
  Top 0.203: IC1.89 50.28,13.33 50.16,13.21 v50.09,13.15 | v42.44,13.14 39.98,15.6 v39.98,17.12 | v22.84,27.28 22.4,26.85 18.06,26.85 17.65,27.25 17.65,29.47 IC5.13
  Bottom 0.203: v50.09,13.15 49.74,13.15 49.72,13.14 42.46,13.14 42.44,13.16 v42.44,13.14 | v39.98,17.12 39.62,17.48 31.98,17.48 22.84,26.62 v22.84,27.28
TCK  (via drill 0.35)
  Top 0.203: IC1.62 39.36,27.93 39.12,27.69 v39.14,27.66 | v29.74,33.71 29.74,34.27 33.38,37.9 v33.38,46.61
  Bottom 0.203: 39.03,27.77 v39.14,27.66 38.79,27.66 38.65,27.52 35.93,27.52 v29.74,33.71 | SV2.1 78.74,42.8 77.47,41.53 72.14,41.53 67.44,46.23 67.44,46.48 41.78,46.48 41.66,46.61 v33.38,46.61
TDI
  Top 0.203: IC1.4 88.19,22.93 88.9,23.64 SV2.9
TDO  (via drill 0.35)
  Top 0.203: IC1.73 40.36,22.43 v40.34,22.45 | v30.2,30.43 34.29,34.52 34.29,45.82 v34.31,45.85
  Bottom 0.203: SV2.3 81.28,44.32 77.85,40.89 71.37,40.89 66.29,45.97 42.55,45.97 42.16,45.85 v34.31,45.85 | v40.34,22.45 38.18,22.45 v30.2,30.43
TMS
  Top 0.203: IC1.15 83.33,28.43 83.82,28.92 SV2.5

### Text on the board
tDocu: LM1030SYR | SPI1 | SERIAL | ATMEL ISP JTAG | Z80 Monsputer bus probe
